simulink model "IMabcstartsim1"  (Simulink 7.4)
settings: Solver=ode45  StartTime=0.0  StopTime=4  MaxStep=1e-3  RelTol=1e-3
InitFcn:
  | imparamstartsim0
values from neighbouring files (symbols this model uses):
  Bm = 0.10    (= 0.1)    [IMabc2.m]    (also in imabcparam.m = 0.01; IMabcrun0.m = 0.01; IMabcrun1.m = 0.001; IMcur0.m = 1e-06)
  D = str2num(get(h,'string'))    [acttrcalc1.m]
  gam = 2*pi/3    (= 2.09439510239)    [IMabc2.m]    (also in IMabcf0.m; IMabcf1.m; imabcparam.m; IMabcrun0.m)
  H = 0.60    (= 0.6)    [IMabc2.m]    (also in IMcur0.m = 0.3; imdef0vec.m = 0.3; imdef1vec.m = 0.3; imdef2vec.m = 0.3)
  Lm1 = 2/3*Lm    [IMabcf0.m]    (also in IMabcf1.m; imabcparam.m = 0.0564666666667; IMabcrun0.m = 0.0564666666667; IMabcrun1.m = 0.0564666666667)
  Lr = Lrl+Lm    (= 4.6)    [IMabc2.m]    (also in IMabcf0.m = Lrl+Lm1; IMabcf1.m = Lrl+Lm1; imabcparam.m = 0.0589666666667; IMcur0.m)
  Ls = Lsl+Lm    (= 4.6)    [IMabc2.m]    (also in IMabcf0.m = Lsl+Lm1; IMabcf1.m = Lsl+Lm1; imabcparam.m = 0.0589666666667; IMcur0.m)
  Rr = input('Rotor resistance)[default = 2] =')    [Actac.m]    (also in im1phase.m = 0.3; im3d.m = eval(get(hRr,'String')); IMabc2.m = 0.02; imabcparam.m = 0.408)
  Rs = eval(get(hRs,'String'))    [im3d.m]    (also in IMabc2.m = 0.01; imabcparam.m = 0.531; IMabcrun0.m = 0.531; IMabcrun1.m = 0.531)
  Vm = Vll*sqrt(2/3)    [imabcparam.m]
  wo = 2*pi*freq0    [calc0.m]    (also in IMabc2.m = 376.991118431; imabcparam.m = 376.991118431; IMabcrun0.m = 376.991118431; IMabcrun1.m = 376.991118431)
undefined symbols (not defined in the file or in its folder): Row, TL1, TL2, vector

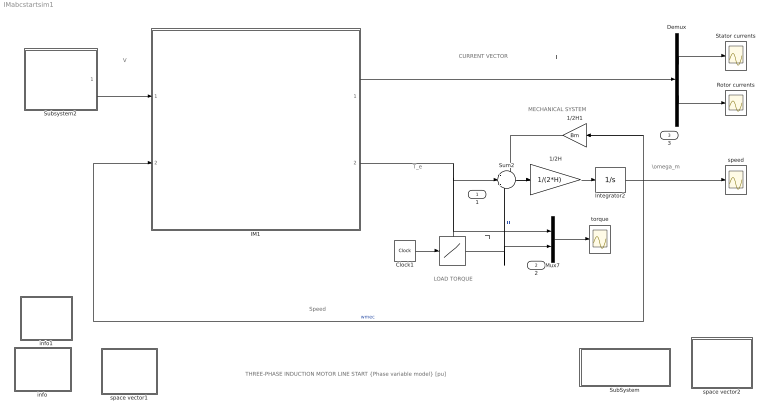
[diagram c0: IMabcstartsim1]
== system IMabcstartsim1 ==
  note: MECHANICAL SYSTEM
  note: \omega_m
  note: THREE-PHASE INDUCTION MOTOR LINE START {Phase variable model} [pu]
  note: TL
  note: LOAD TORQUE
  note: CURRENT VECTOR
  note: I
  note: V
  note: T_e
  note: Speed
  " " : Lookup  InputValues="[0 2 2  4]"  Table="[TL1 TL1  TL2  TL2]"  OutDataType=sfix(16)  OutScaling=2^0
  1/2H : Gain  Gain=1/(2*H)  ParameterDataType=sfix(16)  ParameterScaling=2^0  OutDataType=sfix(16)  OutScaling=2^0
  1/2H1 : Gain  Gain=Bm  ParameterDataType=sfix(16)  ParameterScaling=2^0  OutDataType=sfix(16)  OutScaling=2^0
  Clock1 : Clock
  Demux : Demux  Outputs=2
  IM1 : Subsystem
  Integrator2 : Integrator
  Mux7 : Mux  Inputs=2
  Rotor currents : Scope
  Stator currents : Scope
  SubSystem : Subsystem
  Subsystem2 : Subsystem
  Sum2 : Sum  Inputs=-+-  OutDataType=sfix(16)  OutScaling=2^0
  info : Subsystem
  info1 : Subsystem
  space vector1 : Subsystem
  space vector2 : Subsystem
  speed : Scope
  torque : Scope
  1 : Outport
  2 : Outport  Port=2
  3 : Outport  Port=3
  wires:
  Demux/1 -> Stator currents/1
  Demux/2 -> Rotor currents/1
  Sum2/1 -> 1/2H/1
  1/2H/1 -> Integrator2/1
  Mux7/1 -> torque/1
  " "/1 -> 2/1, Mux7/2, Sum2/3  "TL"
  IM1/2(Te) -> Sum2/2, 1/1, Mux7/1
  Integrator2/1 -> 1/2H1/1, 3/1, speed/1, IM1/2(wm)  "wmec"
  Subsystem2/1(V) -> IM1/1(V)
  Clock1/1 -> " "/1
  1/2H1/1 -> Sum2/1
  IM1/1(I) -> Demux/1

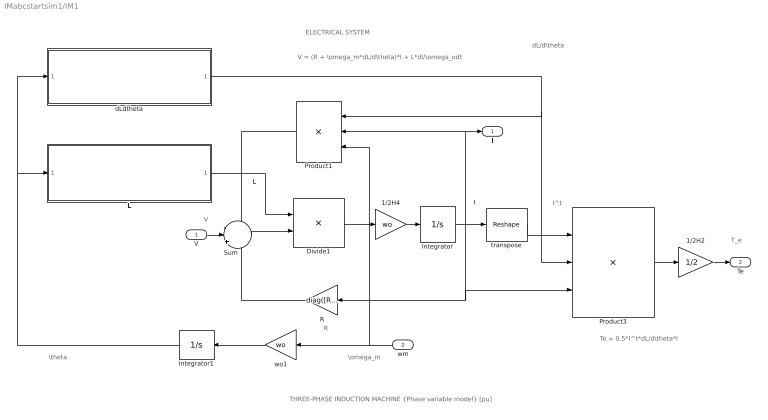
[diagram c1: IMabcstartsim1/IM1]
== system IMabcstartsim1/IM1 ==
  note: I
  note: I^t
  note: ELECTRICAL SYSTEM
  note: V
  note: \theta
  note: L
  note: R
  note: Te = 0.5*I^t*dL/d\theta*I
  note: V = (R + \omega_m*dL/d\theta)*I + L*dI/\omega_odt
  note: dL/d\theta
  note: T_e
  note: \omega_m
  note: THREE-PHASE INDUCTION MACHINE {Phase variable model} [pu]
  V : Inport  OutDataType=sfix(16)  OutScaling=2^0
  wm : Inport  Port=2  OutDataType=sfix(16)  OutScaling=2^0
  1/2H2 : Gain  Gain=1/2  ParameterDataType=sfix(16)  ParameterScaling=2^0  OutDataType=sfix(16)  OutScaling=2^0
  1/2H4 : Gain  Gain=wo  ParameterDataType=sfix(16)  ParameterScaling=2^0  OutDataType=sfix(16)  OutScaling=2^0
  Divide1 : Product  Inputs=/*  Multiplication=Matrix(*)  OutDataType=fixdt(1, 16)  OutScaling=2^-10
  Integrator : Integrator  InitialCondition=[0 ;0 ;0; 0 ;0 ;0]
  Integrator1 : Integrator
  L : Subsystem
  Product1 : Product  Inputs=3  Multiplication=Matrix(*)  OutDataType=fixdt(1, 16)  OutScaling=2^0
  Product3 : Product  Inputs=3  Multiplication=Matrix(*)  OutDataType=sfix(16)  OutScaling=2^0
  R : Gain  Gain=diag([Rs Rs Rs Rr Rr Rr])  Multiplication=Matrix(K*u)  ParameterDataType=sfix(16)  ParameterScaling=2^0  OutDataType=sfix(16)  OutScaling=2^0
  Sum : Sum  Inputs=-|+|-  OutDataType=sfix(16)  OutScaling=2^0
  dLdtheta : Subsystem
  transpose : Reshape  OutputDimensionality=Row vector (2-D)  OutputDimensions=[1,6]
  wo1 : Gain  Gain=wo  ParameterDataType=sfix(16)  ParameterScaling=2^0  OutDataType=sfix(16)  OutScaling=2^0
  I : Outport
  Te : Outport  Port=2
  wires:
  Divide1/1 -> 1/2H4/1
  R/1 -> Sum/3
  transpose/1 -> Product3/1
  Product1/1 -> Sum/1
  dLdtheta/1(dLdtheta) -> Product3/2, Product1/1
  Product3/1 -> 1/2H2/1
  Integrator1/1 -> dLdtheta/1(theta1), L/1(theta)
  L/1(L) -> Divide1/1
  Integrator/1 -> transpose/1, I/1, Product1/2, R/1, Product3/3
  wo1/1 -> Integrator1/1
  1/2H4/1 -> Integrator/1
  wm/1 -> wo1/1, Product1/3
  V/1 -> Sum/2
  1/2H2/1 -> Te/1
  Sum/1 -> Divide1/2

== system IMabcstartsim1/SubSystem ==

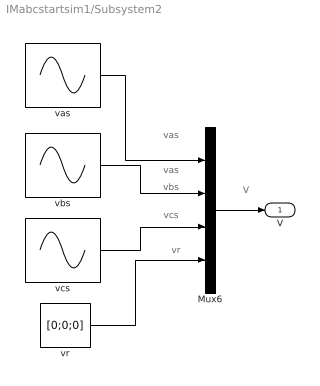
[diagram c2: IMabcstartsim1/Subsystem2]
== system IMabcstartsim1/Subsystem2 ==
  note: vas
  note: vas
  note: vbs
  note: vcs
  note: vr
  note: V
  Mux6 : Mux
  vas : Sin  Amplitude=Vm  Bias=0  Frequency=wo  Phase=pi/2  Samples=10  SampleTime=0
  vbs : Sin  Amplitude=Vm  Bias=0  Frequency=wo  Phase=pi/2-gam  Samples=10  SampleTime=0
  vcs : Sin  Amplitude=Vm  Bias=0  Frequency=wo  Phase=pi/2+gam  Samples=10  SampleTime=0
  vr : Constant  Value=[0;0;0]  VectorParams1D=off  OutDataType=sfix(16)  OutScaling=2^0
  V : Outport
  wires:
  Mux6/1 -> V/1
  vr/1 -> Mux6/4
  vcs/1 -> Mux6/3
  vbs/1 -> Mux6/2
  vas/1 -> Mux6/1

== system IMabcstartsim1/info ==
  note: LINE START OF AN INDUCTION MOTOR (Phase variable model) [pu]
  note: The motor is started by applying three-phase voltages to the stator. The machine dynamic equations are based on a matrix formulation using the phase variables as state variables, namely the stator currents ias, ibs, ics and the rotor currents iar, ibr, icr; the rotor speed wm; and the angular displacement between stator ax_axis and rotor ar_axis. The parameters describing the electromechanical system are expressed in per unit and may be modified by accessing a data file obtained by clicking the PARAMETERS block. The torque developed, the speed, and the stator current are observed on the scopes . The torque-speed dynamic characteristics can then be obtained after double clicking the PLOTS block. To run the identical operation of this motor now formulated in a Matlab script file, run >

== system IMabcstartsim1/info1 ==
  note: This demonstration illustrates the dynamics of a synchronous generator, initially at no load, following a three-phase short circuit at the terminals.
  note: Synchronous machine transients under shortcircuit

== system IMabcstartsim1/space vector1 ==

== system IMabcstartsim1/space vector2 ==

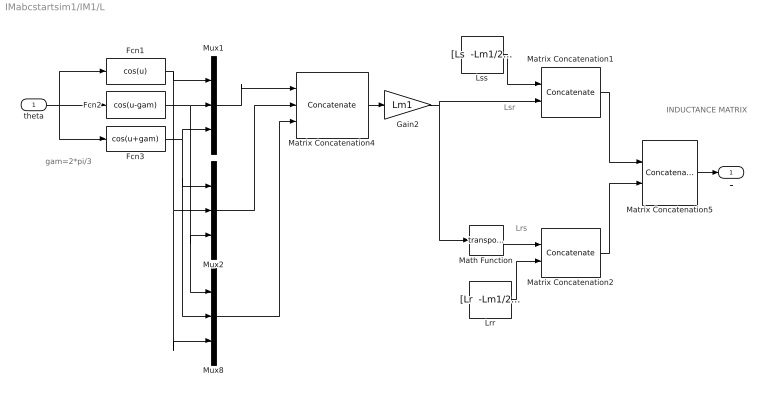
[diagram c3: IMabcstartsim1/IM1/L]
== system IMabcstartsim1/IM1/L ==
  note: Lrs
  note: Lsr
  note: INDUCTANCE MATRIX
  note: gam=2*pi/3
  theta : Inport  OutDataType=sfix(16)  OutScaling=2^0
  Fcn1 : Fcn  Expr=cos(u)
  Fcn2 : Fcn  Expr=cos(u-gam)
  Fcn3 : Fcn  Expr=cos(u+gam)
  Gain2 : Gain  Gain=Lm1  ParameterDataType=sfix(16)  ParameterScaling=2^0  OutDataType=sfix(16)  OutScaling=2^0
  Lrr : Constant  Value="[Lr  -Lm1/2  -Lm1/2; -Lm1/2  Lr -Lm1/2;-Lm1/2  -Lm1/2  Lr]"  VectorParams1D=off  OutDataType=sfix(16)  OutScaling=2^0
  Lss : Constant  Value="[Ls  -Lm1/2  -Lm1/2; -Lm1/2  Ls  -Lm1/2;-Lm1/2  -Lm1/2  Ls]"  VectorParams1D=off  OutDataType=sfix(16)  OutScaling=2^0
  Math Function : Math  Operator=transpose
  Matrix Concatenation1 : Concatenate  Mode=Multidimensional array  ConcatenateDimension=2
  Matrix Concatenation2 : Concatenate  Mode=Multidimensional array  ConcatenateDimension=2
  Matrix Concatenation4 : Concatenate  NumInputs=3  Mode=Multidimensional array  ConcatenateDimension=2
  Matrix Concatenation5 : Concatenate  Mode=Multidimensional array
  Mux1 : Mux  Inputs=3
  Mux2 : Mux  Inputs=3
  Mux8 : Mux  Inputs=3
  L : Outport
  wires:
  Fcn1/1 -> Mux1/1, Mux2/2, Mux8/3
  Fcn2/1 -> Mux8/1, Mux2/3, Mux1/2
  Fcn3/1 -> Mux8/2, Mux2/1, Mux1/3
  Lrr/1 -> Matrix Concatenation2/2
  Lss/1 -> Matrix Concatenation1/1
  Matrix Concatenation2/1 -> Matrix Concatenation5/2
  Matrix Concatenation1/1 -> Matrix Concatenation5/1
  Mux2/1 -> Matrix Concatenation4/2
  Mux8/1 -> Matrix Concatenation4/3
  Matrix Concatenation4/1 -> Gain2/1
  Mux1/1 -> Matrix Concatenation4/1
  Gain2/1 -> Math Function/1, Matrix Concatenation1/2
  Math Function/1 -> Matrix Concatenation2/1
  theta/1 -> Fcn2/1, Fcn1/1, Fcn3/1
  Matrix Concatenation5/1 -> L/1

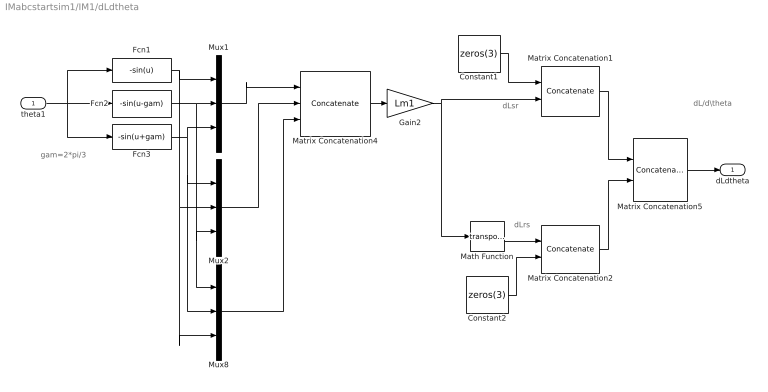
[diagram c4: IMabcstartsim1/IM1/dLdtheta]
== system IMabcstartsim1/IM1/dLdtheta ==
  note: dLrs
  note: dLsr
  note: dL/d\theta
  note: gam=2*pi/3
  theta1 : Inport  OutDataType=sfix(16)  OutScaling=2^0
  Constant1 : Constant  Value=zeros(3)  VectorParams1D=off  OutDataType=sfix(16)  OutScaling=2^0
  Constant2 : Constant  Value=zeros(3)  VectorParams1D=off  OutDataType=sfix(16)  OutScaling=2^0
  Fcn1 : Fcn  Expr=-sin(u)
  Fcn2 : Fcn  Expr=-sin(u-gam)
  Fcn3 : Fcn  Expr=-sin(u+gam)
  Gain2 : Gain  Gain=Lm1  ParameterDataType=sfix(16)  ParameterScaling=2^0  OutDataType=sfix(16)  OutScaling=2^0
  Math Function : Math  Operator=transpose
  Matrix Concatenation1 : Concatenate  Mode=Multidimensional array  ConcatenateDimension=2
  Matrix Concatenation2 : Concatenate  Mode=Multidimensional array  ConcatenateDimension=2
  Matrix Concatenation4 : Concatenate  NumInputs=3  Mode=Multidimensional array  ConcatenateDimension=2
  Matrix Concatenation5 : Concatenate  Mode=Multidimensional array
  Mux1 : Mux  Inputs=3
  Mux2 : Mux  Inputs=3
  Mux8 : Mux  Inputs=3
  dLdtheta : Outport
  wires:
  Matrix Concatenation5/1 -> dLdtheta/1
  Fcn1/1 -> Mux1/1, Mux2/2, Mux8/3
  Fcn2/1 -> Mux8/1, Mux2/3, Mux1/2
  Fcn3/1 -> Mux8/2, Mux2/1, Mux1/3
  Constant2/1 -> Matrix Concatenation2/2
  Constant1/1 -> Matrix Concatenation1/1
  Matrix Concatenation2/1 -> Matrix Concatenation5/2
  Matrix Concatenation1/1 -> Matrix Concatenation5/1
  Mux2/1 -> Matrix Concatenation4/2
  Mux8/1 -> Matrix Concatenation4/3
  Matrix Concatenation4/1 -> Gain2/1
  Mux1/1 -> Matrix Concatenation4/1
  Gain2/1 -> Math Function/1, Matrix Concatenation1/2
  Math Function/1 -> Matrix Concatenation2/1
  theta1/1 -> Fcn3/1, Fcn2/1, Fcn1/1
